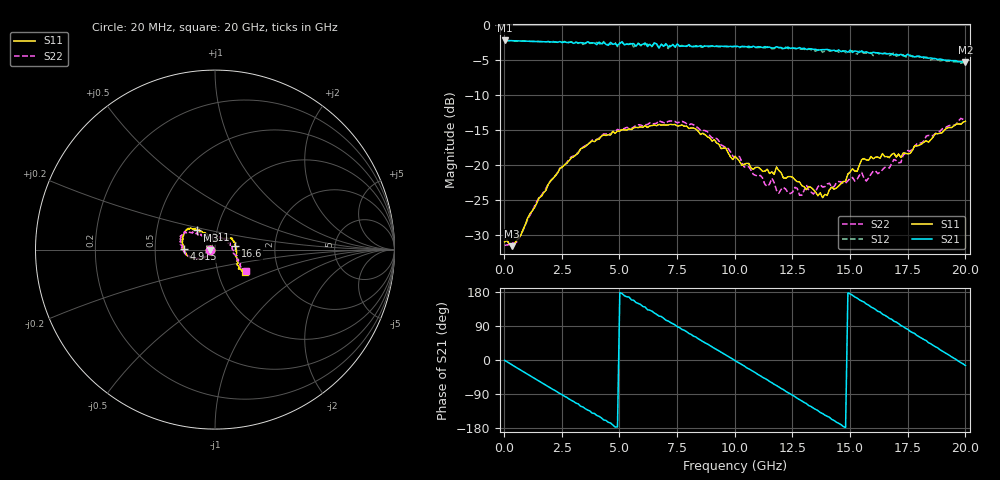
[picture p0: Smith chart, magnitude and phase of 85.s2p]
!Agilent Technologies,N5230A,US43500223,A.07.50.48
!Agilent N5230A: A.07.50.48
!Date: Saturday, September 19, 2015 17:11:11
!Correction: S11(Full 2 Port(1,2))
!S21(Full 2 Port(1,2))
!S12(Full 2 Port(1,2))
!S22(Full 2 Port(1,2))
!S2P File: Measurements: S11, S21, S12, S22:
# Hz S  dB  R 50
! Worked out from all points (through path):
!   201 points, 20 MHz to 20 GHz, reference 50 ohm
!   highest |S21| = -2.16 dB at 20 MHz (marker M1); lowest = -5.3 dB at 20 GHz (marker M2)
!   group delay of S21, straight-line fit = 102 ps
!   lowest |S11| = -31.6 dB at 319.7 MHz (marker M3), VSWR 1.05, Z = 47.5 - j0.45 ohm
!   |S11| at or under -10 dB: start of sweep to end of sweep
!   |S22| runs from -31.5 to -13.3 dB; largest |S21 - S12| = 0.043
!   S11 on the Smith chart (normalised r, x): 20 MHz: 0.94, -0.00; 4.915 GHz: 0.70, +0.00; 9.011 GHz: 0.80, +0.18; 16.6 GHz: 1.25, +0.05; 20 GHz: 1.34, -0.35
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2e7  -30.97 -178.8  -2.16 -0.8  -2.16 -0.8  -31.47 178.9
3.197e8  -31.58 -169.6  -2.20 -12.0  -2.20 -12.0  -31.13 -170.1
1.9181e9  -22.70 -143.0  -2.31 -70.4  -2.31 -70.5  -22.64 -143.5
2.6174e9  -19.95 -149.5  -2.35 -95.9  -2.29 -96.1  -19.99 -149.8
3.4166e9  -17.52 -158.9  -2.50 -123.9  -2.72 -124.2  -17.41 -159.2
4.3157e9  -15.66 -169.9  -2.45 -158.3  -2.31 -156.2  -15.52 -172.0
4.9151e9  -15.12 179.3  -2.87 -176.5  -3.05 -177.3  -14.88 -178.7
5.8142e9  -14.63 166.3  -2.59 149.2  -2.54 149.7  -14.21 171.8
6.7133e9  -14.16 155.1  -3.24 115.9  -3.20 116.3  -13.62 162.8
7.5125e9  -14.40 146.2  -2.66 87.6  -2.83 89.6  -13.95 156.2
9.011e9  -16.55 133.3  -2.92 34.8  -2.98 35.4  -16.11 143.2
1.001e10  -18.72 125.9  -3.01 -1.6  -3.00 -1.2  -18.93 132.6
1.08092e10  -20.58 121.3  -2.98 -30.4  -3.08 -30.1  -21.33 127.9
1.18082e10  -20.26 118.9  -3.05 -67.4  -3.09 -66.8  -23.58 110.4
1.26074e10  -22.10 112.3  -3.29 -96.6  -3.30 -97.0  -23.17 105.0
1.34066e10  -23.46 98.1  -3.42 -126.8  -3.50 -127.5  -24.11 91.6
1.5005e10  -20.96 45.7  -3.54 174.5  -3.83 177.0  -21.87 53.2
1.66034e10  -18.76 10.2  -4.10 114.5  -4.03 113.8  -20.33 6.8
1.67033e10  -18.91 12.5  -4.03 109.7  -4.32 111.8  -20.39 0.9
1.79021e10  -17.24 -26.3  -4.42 64.7  -4.40 67.3  -16.94 -23.6
1.88012e10  -15.50 -37.5  -4.90 31.9  -4.86 31.1  -15.30 -34.2
2e10  -13.72 -36.8  -5.26 -14.7  -5.36 -13.7  -13.64 -34.6
